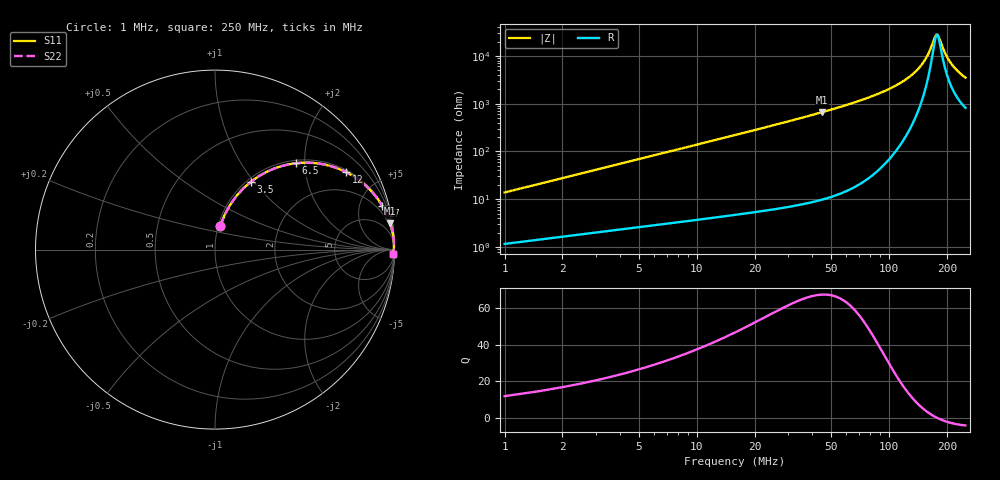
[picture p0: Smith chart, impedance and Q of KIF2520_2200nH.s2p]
!version-2
!date-12.2020
!Series
# MHz S RI R 50
!Freq ReS11 ImS11 ReS21 ImS21 ReS12 ImS12 ReS22 ImS22
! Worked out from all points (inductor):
!   499 points, 1 MHz to 250 MHz, reference 50 ohm
!   read as one part in series: L = 2.2 uH near 2 MHz
!   highest Q = 67.5 at 45 MHz (marker M1), where L = 2.35 uH
!   self-resonance near 178 MHz
!   S11 on the Smith chart (normalised r, x): 1 MHz: 1.02, +0.28; 3.5 MHz: 1.04, +0.97; 6.5 MHz: 1.06, +1.80; 12 MHz: 1.08, +3.33; 27 MHz: 1.13, +7.64; 250 MHz: 17, -68
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1  0.0296 0.1326  0.9704 -0.1326  0.9704 -0.1326  0.0296 0.1326
2.5  0.1195 0.2989  0.8805 -0.2989  0.8805 -0.2989  0.1195 0.2989
3.5  0.2007 0.3786  0.7993 -0.3786  0.7993 -0.3786  0.2007 0.3786
5  0.3299 0.4517  0.6701 -0.4517  0.6701 -0.4517  0.3299 0.4517
6.5  0.4493 0.4812  0.5507 -0.4812  0.5507 -0.4812  0.4493 0.4812
9  0.606 0.4748  0.394 -0.4748  0.394 -0.4748  0.606 0.4748
12  0.7304 0.4317  0.2696 -0.4317  0.2696 -0.4317  0.7304 0.4317
18  0.8585 0.3386  0.1415 -0.3386  0.1415 -0.3386  0.8585 0.3386
27  0.9323 0.2429  0.0677 -0.2429  0.0677 -0.2429  0.9323 0.2429
42.5  0.9727 0.1557  0.0273 -0.1557  0.0273 -0.1557  0.9727 0.1557
45  0.9758 0.1465  0.0242 -0.1465  0.0242 -0.1465  0.9758 0.1465
84  0.994 0.0664  0.00596 -0.0664  0.00596 -0.0664  0.994 0.0664
125.5  0.9971 0.0288  0.00291 -0.0288  0.00291 -0.0288  0.9971 0.0288
150  0.9971 0.0139  0.00287 -0.0139  0.00287 -0.0139  0.9971 0.0139
159  0.997 0.00917  0.00302 -0.00917  0.00302 -0.00917  0.997 0.00917
167  0.9968 0.00521  0.00322 -0.00521  0.00322 -0.00521  0.9968 0.00521
174.5  0.9966 0.00168  0.00344 -0.00168  0.00344 -0.00168  0.9966 0.00168
179  0.9964 -0.00036  0.00359 0.00036  0.00359 0.00036  0.9964 -0.00036
195.5  0.9958 -0.00741  0.00425 0.00741  0.00425 0.00741  0.9958 -0.00741
208.5  0.9951 -0.0126  0.00487 0.0126  0.00487 0.0126  0.9951 -0.0126
227  0.9941 -0.0194  0.00589 0.0194  0.00589 0.0194  0.9941 -0.0194
250  0.9927 -0.0273  0.00735 0.0273  0.00735 0.0273  0.9927 -0.0273
